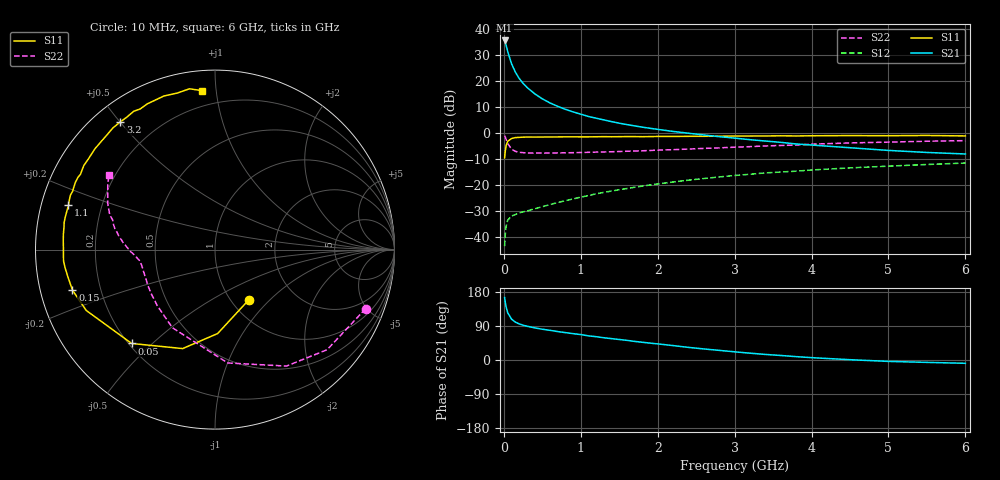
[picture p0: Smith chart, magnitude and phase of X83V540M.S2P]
! SIEMENS Small Signal Semiconductors
! BFP136W
! Si NPN RF Bipolar Junction Transistor in SOT343
! VCE = 3.5 V  IC = 40 mA
! Common Emitter S-Parameters:  September  1994
# GHz  S  MA  R  50
!  f  S11  S21  S12  S22
! GHz  MAG  ANG  MAG  ANG  MAG  ANG  MAG  ANG
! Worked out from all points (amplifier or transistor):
!   40 points, 10 MHz to 6 GHz, reference 50 ohm
!   highest |S21| = 35.6 dB at 10 MHz (marker M1)
!   |S21| within 3 dB of that: start of sweep to 39.45 MHz
!   unconditionally stable (mu >= 1): 705.5 MHz to 2.852 GHz
!   at 200 MHz: K = 0.49, MSG = 25.8 dB, |S12| = -30.6 dB
!   at 1.5 GHz: K = 1.11, MAG = 10.7 dB, |S12| = -21.7 dB
!   at 6 GHz: K = 0.97, MSG = 1.7 dB, |S12| = -11.4 dB
!   S11 on the Smith chart (normalised r, x): 10 MHz: 1.20, -0.76; 50 MHz: 0.21, -0.43; 150 MHz: 0.10, -0.14; 1.1 GHz: 0.08, +0.15; 3.2 GHz: 0.08, +0.50; 6 GHz: 0.11, +0.92
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0.01  0.3372 -56.0  60.44 164.6  0.0068 74.5  0.9017 -21.4
0.02  0.4679 -88.2  54.55 150.8  0.0121 64.5  0.8373 -41.8
0.03  0.5802 -108.1  48.66 139.9  0.0165 53.5  0.7611 -58.5
0.05  0.6994 -131.6  37.06 124.9  0.0214 41.2  0.6356 -83.6
0.1  0.7935 -154.7  21.6 107.8  0.0258 32.0  0.4961 -118.5
0.15  0.8256 -164.1  14.9 99.9  0.0275 30.5  0.449 -135.6
0.2  0.8332 -169.3  11.24 95.2  0.0296 32.1  0.4318 -145.5
0.25  0.8414 -173.1  9.09 91.8  0.031 33.3  0.4241 -151.8
0.3  0.8463 -175.8  7.613 89.2  0.0322 34.7  0.4188 -156.1
0.4  0.8445 179.7  5.74 84.8  0.0355 39.0  0.4163 -161.7
0.5  0.8468 176.7  4.575 81.2  0.0389 42.3  0.4164 -165.2
0.6  0.8492 174.1  3.817 78.3  0.0428 45.0  0.4176 -167.4
0.7  0.8505 171.6  3.289 75.0  0.0467 47.9  0.419 -168.9
0.9  0.8537 167.7  2.572 69.5  0.0549 51.1  0.4239 -171.4
1.1  0.8529 163.2  2.102 63.7  0.0637 53.2  0.4308 -172.9
1.4  0.8573 157.9  1.672 56.4  0.0777 54.9  0.4415 -174.8
1.6  0.8635 154.2  1.467 51.8  0.0869 55.0  0.4516 -176.3
2.2  0.8679 143.9  1.084 38.0  0.116 53.4  0.4839 179.4
3.2  0.8856 126.6  0.752 18.0  0.1633 46.2  0.5536 170.1
4.5  0.9019 108.4  0.527 0.8  0.2164 34.6  0.6517 156.6
5.5  0.9072 99.0  0.428 -6.3  0.2512 26.7  0.7029 148.2
6  0.8879 94.5  0.4 -8.7  0.2682 22.3  0.7218 144.7
